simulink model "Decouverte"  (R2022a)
settings: Solver=VariableStepAuto  StartTime=0.0  StopTime=inf  RelTol=1e-3
libraries: fl_lib x15, nesl_utility x6

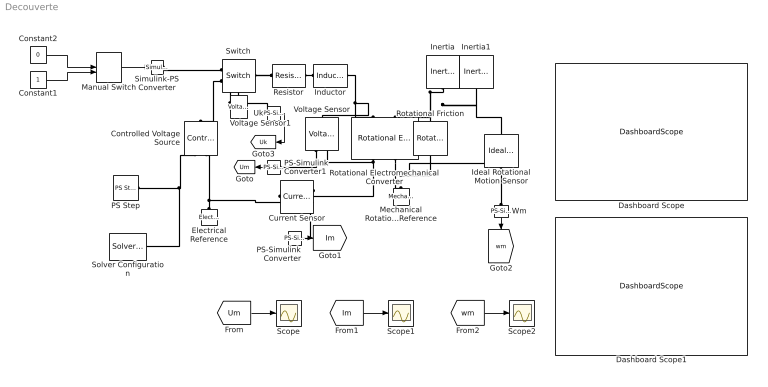
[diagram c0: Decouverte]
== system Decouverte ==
  Constant1 : Constant
  Constant2 : Constant  Value=0
  Controlled Voltage Source : fl_lib/Electrical/Electrical Sources/Controlled Voltage Source
  Current Sensor : fl_lib/Electrical/Electrical Sensors/Current Sensor
  Dashboard Scope : DashboardScope  Ymin=0  Ymax=1500  ScaleAtStop=off
  Dashboard Scope1 : DashboardScope  Ymin=0  Ymax=14  ScaleAtStop=off
  Electrical Reference : fl_lib/Electrical/Electrical Elements/Electrical Reference
  Ideal Rotational Motion Sensor : fl_lib/Mechanical/Mechanical Sensors/Ideal Rotational Motion Sensor  wrap_angle=simscape.enum.onoff.off  offset=0 rad
  Inductor : fl_lib/Electrical/Electrical Elements/Inductor  l=0.004 H  r=0 Ohm  g=1e-9 1/Ohm  i_specify=off  i_priority=None  i=0 A  i_nominal_specify=off  i_nominal_unit=A  i_nominal_value=1  v_specify=off  v_priority=None  v=0 V  v_nominal_specify=off  v_nominal_unit=V  v_nominal_value=1  i_L_specify=off  i_L_priority=High  i_L=0 A  i_L_nominal_specify=off  i_L_nominal_unit=A  i_L_nominal_value=1
  Inertia : fl_lib/Mechanical/Rotational Elements/Inertia  inertia=3e-6 kg*m^2  num_ports=foundation.enum.numPorts2.one  w_specify=off  w_priority=High  w=0 rad/s  w_nominal_specify=off  w_nominal_unit=rad/s  w_nominal_value=1  t_specify=off  t_priority=None  t=0 N*m  t_nominal_specify=off  t_nominal_unit=N*m  t_nominal_value=1
  Inertia1 : fl_lib/Mechanical/Rotational Elements/Inertia  inertia=0.0001 kg*m^2  num_ports=foundation.enum.numPorts2.one  w_specify=off  w_priority=High  w=0 rad/s  w_nominal_specify=off  w_nominal_unit=rad/s  w_nominal_value=1  t_specify=off  t_priority=None  t=0 N*m  t_nominal_specify=off  t_nominal_unit=N*m  t_nominal_value=1
  Manual Switch : ManualSwitch  CurrentSetting=0
  Mechanical Rotational Reference : fl_lib/Mechanical/Rotational Elements/Mechanical Rotational Reference
  PS Step : fl_lib/Physical Signals/Sources/PS Step  step_time=0 s  initial_value=0  final_value=12
  PS-Simulink Converter : nesl_utility/PS-Simulink Converter  PhysicalDomain=network_engine_domain  SubClassName=ps_output  LeftPortType=input  RightPortType=output  PseudoPeriodic=off  Frequencies=[]  VectorFormat=1-D array  Unit=inherit  AffineConversion=off
  PS-Simulink Converter1 : nesl_utility/PS-Simulink Converter  PhysicalDomain=network_engine_domain  SubClassName=ps_output  LeftPortType=input  RightPortType=output  PseudoPeriodic=off  Frequencies=[]  VectorFormat=1-D array  Unit=inherit  AffineConversion=off
  Resistor : fl_lib/Electrical/Electrical Elements/Resistor  R=3 Ohm  i_specify=off  i_priority=None  i=0 A  i_nominal_specify=off  i_nominal_unit=A  i_nominal_value=1  v_specify=off  v_priority=None  v=0 V  v_nominal_specify=off  v_nominal_unit=V  v_nominal_value=1
  Rotational Electromechanical Converter : fl_lib/Electrical/Electrical Elements/Rotational Electromechanical Converter  K=0.009 V*s/rad  i_specify=off  i_priority=None  i=0 A  i_nominal_specify=off  i_nominal_unit=A  i_nominal_value=1  v_specify=off  v_priority=None  v=0 V  v_nominal_specify=off  v_nominal_unit=V  v_nominal_value=1  t_specify=off  t_priority=None  t=0 N*m  t_nominal_specify=off  t_nominal_unit=N*m  t_nominal_value=1  w_specify=off  w_priority=None  w=0 rad/s  w_nominal_specify=off  w_nominal_unit=rad/s  w_nominal_value=1
  Rotational Friction : fl_lib/Mechanical/Rotational Elements/Rotational Friction  brkwy_trq=0.0000000001 N*m  brkwy_vel=0.0000000001 rad/s  Col_trq=0.0000000001 N*m  visc_coef=0.0000025 N*m/(rad/s)  w_specify=off  w_priority=None  w=0 rad/s  w_nominal_specify=off  w_nominal_unit=rad/s  w_nominal_value=1  t_specify=off  t_priority=None  t=0 N*m  t_nominal_specify=off  t_nominal_unit=N*m  t_nominal_value=1
  Scope : Scope
  Scope1 : Scope
  Scope2 : Scope
  Simulink-PS Converter : nesl_utility/Simulink-PS Converter  PhysicalDomain=network_engine_domain  SubClassName=ps_input  LeftPortType=input  RightPortType=output  PseudoPeriodic=off  Frequencies=[]  NoiseDistribution=none  NoiseParameters=[]  Unit=1  AffineConversion=off  FilteringAndDerivatives=provide  SimscapeFilterOrder=1  InputFilterTimeConstant=0.001  UdotUserProvided=0
  Solver Configuration : nesl_utility/Solver Configuration  PhysicalDomain=network_engine_domain  SubClassName=solver  LeftPortType=input  RightPortType=generic  Tones=[]  Harmonics=[]  SimulateNoise=off  Profile=off  UseLocalSampling=off  EnableSwitchedLinearOptims=on  FrequencyDomain=off  UseCCode=off  RelTol=0.001  AbsTol=1e-06  MinStep=1e-09  ToWorkspace=off  RevertToSquareIcSolve=off  NumHomotopyIterations=100  PhasorMode=off  PhasorModeNumHarmonics=1  IndexReductionMethod=DerivativeReplacement  DoDC=off  ResidualTolerance=1e-09  UseLocalSolver=off  LocalSolverChoice=NE_BACKWARD_EULER_ADVANCER  LocalSolverSampleTime=0.001  DoFixedCost=off  MaxNonlinIter=3  MaxModeIter=2  ComputeImpulses=off  ImpulseIterations=2  LinearAlgebra=auto  LinearAlgebraNumThread=0  EquationFormulation=NE_TIME_EF  DelaysMemoryBudget=1024  AutomaticFiltering=on  FilteringTimeConstant=0.001  PartitionStorageMethod=AS_NEEDED  PartitionMemoryBudget=1024  PartitionMethod=ROBUST
  Switch : fl_lib/Electrical/Electrical Elements/Switch  R_closed=0.0001 Ohm  G_open=1e-8 1/Ohm  Threshold=0.5  i_specify=off  i_priority=None  i=0 A  i_nominal_specify=off  i_nominal_unit=A  i_nominal_value=1  v_specify=off  v_priority=None  v=0 V  v_nominal_specify=off  v_nominal_unit=V  v_nominal_value=1
  Uk : nesl_utility/PS-Simulink Converter  PhysicalDomain=network_engine_domain  SubClassName=ps_output  LeftPortType=input  RightPortType=output  PseudoPeriodic=off  Frequencies=[]  VectorFormat=1-D array  Unit=inherit  AffineConversion=off
  Voltage Sensor : fl_lib/Electrical/Electrical Sensors/Voltage Sensor
  Voltage Sensor1 : fl_lib/Electrical/Electrical Sensors/Voltage Sensor
  Wm : nesl_utility/PS-Simulink Converter  PhysicalDomain=network_engine_domain  SubClassName=ps_output  LeftPortType=input  RightPortType=output  PseudoPeriodic=off  Frequencies=[]  VectorFormat=1-D array  Unit=inherit  AffineConversion=off
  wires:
  PS-Simulink Converter1/1 -> [Um]
  PS-Simulink Converter/1 -> [Im]
  [Um] -> Scope/1
  [Im] -> Scope1/1
  Wm/1 -> [wm]
  [wm] -> Scope2/1
  Manual Switch/1 -> Simulink-PS Converter/1
  Constant2/1 -> Manual Switch/1
  Constant1/1 -> Manual Switch/2
  Uk/1 -> [Uk]
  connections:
  PS Step/RConn1 -- Solver Configuration/RConn1 -- Controlled Voltage Source/RConn1
  Electrical Reference/LConn1 -- Controlled Voltage Source/RConn2 -- Current Sensor/RConn2
  Resistor/RConn1 -- Inductor/LConn1
  Inductor/RConn1 -- Voltage Sensor/LConn1 -- Rotational Electromechanical Converter/LConn1
  Resistor/LConn1 -- Voltage Sensor1/RConn2 -- Switch/LConn1
  Switch/RConn2 -- Voltage Sensor1/LConn1 -- Controlled Voltage Source/LConn1
  Rotational Electromechanical Converter/RConn2 -- Rotational Friction/RConn1 -- Ideal Rotational Motion Sensor/RConn1 -- Mechanical Rotational Reference/LConn1
  Inertia/LConn1 -- Inertia1/LConn1 -- Ideal Rotational Motion Sensor/LConn1 -- Rotational Electromechanical Converter/LConn2 -- Rotational Friction/LConn1
  Rotational Electromechanical Converter/RConn1 -- Voltage Sensor/RConn2 -- Current Sensor/LConn1
  Voltage Sensor/RConn1 -- PS-Simulink Converter1/LConn1
  Current Sensor/RConn1 -- PS-Simulink Converter/LConn1
  Wm/LConn1 -- Ideal Rotational Motion Sensor/RConn2
  Simulink-PS Converter/RConn1 -- Switch/RConn1
  Uk/LConn1 -- Voltage Sensor1/RConn1
